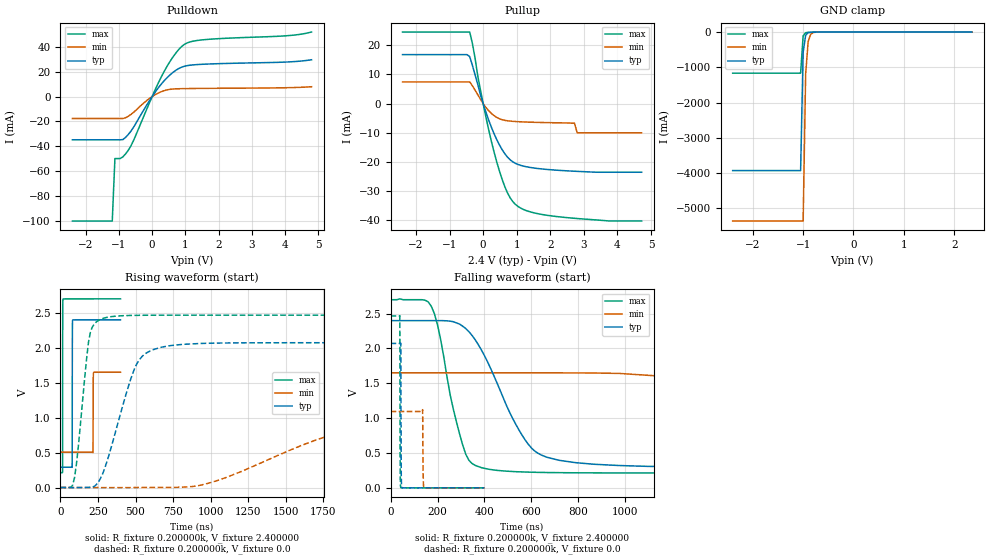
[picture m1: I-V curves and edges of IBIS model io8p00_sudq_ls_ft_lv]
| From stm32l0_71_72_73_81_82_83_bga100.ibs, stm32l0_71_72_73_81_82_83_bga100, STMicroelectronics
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|   Model io8p00_sudq_ls_ft_lv
[Model]  io8p00_sudq_ls_ft_lv
Model_type I/O
Polarity   Non-Inverting
Enable   Active-Low
Vinl =   0.720000V
Vinh =   1.680000V
Vmeas =  1.200000V
Cref =   50.000000pF
Rref =   100.000000M
Vref =   0.0V
C_comp   2.317700pF   2.286600pF   2.332700pF
[Temperature Range]   25.000000   0.105000k   -40.000000
[Pullup Reference]   2.400000V   1.650000V   2.700000V
[Pulldown Reference]   0.0V   0.0V   0.0V
[POWER Clamp Reference]   2.400000V   1.650000V   2.700000V
[GND Clamp Reference]   0.0V   0.0V   0.0V
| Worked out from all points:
|   slope of the pulldown table from 0 to 0.36 V, typ, clamps not added: 28.4 ohm
|   slope of the pullup table from 0 to 0.36 V, typ, clamps not added: 32.2 ohm
|   GND clamp passes 1 mA (typ) near -0.65 V on its own axis
|   rising waveform, R_fixture 0.200000k, V_fixture 2.400000: 20-80 % time 640ps typ, 835ps min, 684ps max; typ from 0.291 V to 2.4 V
|   rising waveform, R_fixture 0.200000k, V_fixture 0.0: 20-80 % time 170ns typ, 822ns min, 66.7ns max; typ from 0 V to 2.07 V
|   falling waveform, R_fixture 0.200000k, V_fixture 2.400000: 20-80 % time 182ns typ, 733ns min, 90.7ns max; typ from 2.4 V to 0.291 V
|   falling waveform, R_fixture 0.200000k, V_fixture 0.0: 20-80 % time 1.11ns typ, 1.65ns min, 899ps max; typ from 2.07 V to 0 V
[Pulldown]
|Voltage   I(typ)   I(min)   I(max)
-2.4V     -34.7mA    -17.61mA   -100mA
-1.2V     -34.7mA    -17.61mA   -100mA
-1.12V    -34.7mA    -17.61mA   -49.77mA
-960mV    -34.7mA    -17.61mA   -49.77mA
-720mV    -30.52mA   -15.81mA   -43.24mA
-560mV    -24.66mA   -12.69mA   -35.31mA
-80mV     -3.3mA     -1.497mA   -4.982mA
320mV     11.47mA    4.39mA     18.08mA
640mV     19.72mA    6.139mA    32.34mA
960mV     24.32mA    6.432mA    41.77mA
1.52V     26.01mA    6.612mA    45.64mA
4.8V      29.64mA    7.944mA    51.92mA
[Pullup]
|Voltage   I(typ)   I(min)   I(max)
-2.4V     16.77mA    7.419mA    24.51mA
-400mV    16.1mA     7.419mA    24.51mA
-320mV    13.11mA    6.112mA    20.64mA
-160mV    6.585mA    3.046mA    9.467mA
80mV      -2.838mA   -1.261mA   -4.478mA
400mV     -12.2mA    -4.699mA   -19.76mA
720mV     -18.26mA   -5.869mA   -30.44mA
1.04V     -20.85mA   -6.184mA   -35.23mA
1.6V      -22.18mA   -6.425mA   -37.62mA
2.72V     -23.16mA   -6.7mA     -39.27mA
2.8V      -23.2mA    -10mA      -39.35mA
4.72V     -23.5mA    -10mA      -40.2mA
[GND_clamp]
|Voltage   I(typ)   I(min)   I(max)
-2.4V     -3.929A    -5.359A    -1.166A
-1.05V    -3.929A    -5.359A    -1.166A
-1V       -574.5mA   -5.359A    -109.1mA
-950mV    -90.02mA   -1.192A    -18.55mA
-900mV    -18.41mA   -269.7mA   -9.049mA
-850mV    -6.764mA   -63.59mA   -6.579mA
-800mV    -4.027mA   -16.66mA   -4.859mA
-650mV    -1.043mA   -1.218mA   -1.146mA
2.35V     0A         0A         0A
[POWER_clamp]
|Voltage   I(typ)   I(min)   I(max)
-2.4V     0A         0A         0A
0V        0A         0A         0A
[Ramp]
| variable   typ   min   max
dV/dt_r  0.65070/0.30307u   0.18995/0.81921u   1.03800/0.14417u
dV/dt_f  0.75696/0.32398u   0.19686/0.85217u   1.13786/0.16139u
R_load = 50.000000
[Rising Waveform]
R_fixture= 0.200000k
V_fixture= 2.400000
V_fixture_min= 1.650000
V_fixture_max= 2.700000
|time   V(typ)   V(min)   V(max)
0s        290.7mV    506.7mV    213mV
14.01ns   290.7mV    506.7mV    219.9mV
15.22ns   290.7mV    506.7mV    2.493V
17.22ns   290.7mV    506.7mV    2.696V
77.68ns   288.9mV    506.7mV    2.7V
79.28ns   2.132V     506.7mV    2.7V
81.28ns   2.395V     506.7mV    2.7V
215.8ns   2.4V       498.8mV    2.7V
220.6ns   2.4V       1.646V     2.7V
400ns     2.4V       1.65V      2.7V
[Rising Waveform]
R_fixture= 0.200000k
V_fixture= 0.0
V_fixture_min= 0.0
V_fixture_max= 0.0
|time   V(typ)   V(min)   V(max)
0s        1.73nV     10.51nV    1.322nV
93.43ns   -108.5uV   10.51nV    137.6mV
200.2ns   3.641mV    10.52nV    2.232V
280.3ns   192.8mV    -23.12uV   2.417V
373.7ns   852.2mV    -23.26uV   2.454V
547.2ns   1.884V     275uV      2.465V
934.3ns   2.062V     34.58mV    2.467V
1.975us   2.072V     857.2mV    2.467V
2.763us   2.072V     1.058V     2.467V
13.33us   2.072V     1.095V     2.467V
[Falling Waveform]
R_fixture= 0.200000k
V_fixture= 2.400000
V_fixture_min= 1.650000
V_fixture_max= 2.700000
|time   V(typ)   V(min)   V(max)
0s        2.4V       1.65V      2.7V
173.5ns   2.4V       1.65V      2.607V
320.3ns   2.286V     1.65V      483.1mV
533.9ns   910.5mV    1.65V      231.9mV
640.6ns   473.9mV    1.65V      221.6mV
867.5ns   338.4mV    1.648V     214.9mV
1.348us   297.4mV    1.506V     213mV
2.229us   290.8mV    716mV      213mV
3.083us   290.7mV    544.2mV    213mV
13.33us   290.7mV    506.7mV    213mV
[Falling Waveform]
R_fixture= 0.200000k
V_fixture= 0.0
V_fixture_min= 0.0
V_fixture_max= 0.0
|time   V(typ)   V(min)   V(max)
0s        2.072V     1.095V     2.467V
39.24ns   2.072V     1.095V     2.471V
40.84ns   2.072V     1.095V     335.4mV
43.64ns   2.071V     1.095V     3.507mV
45.25ns   328.6mV    1.095V     939.5uV
48.05ns   4.133mV    1.095V     306.7uV
136.5ns   18.4uV     1.121V     133.7uV
138.9ns   18.54uV    197.8mV    134.1uV
142.5ns   18.74uV    3.856mV    134.6uV
400ns     1.73nV     10.51nV    1.322nV
